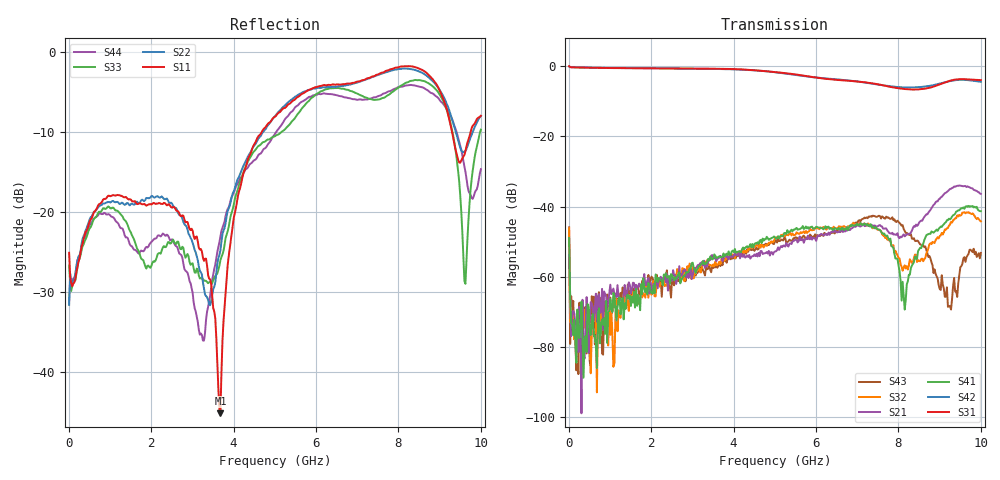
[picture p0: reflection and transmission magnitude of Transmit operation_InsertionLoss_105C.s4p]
! Device:  ADRF5545A
! Description: Dual-Channel, Receiver Front End
! Frequency:  2.4 -  4.2 GHz
! Ports:
!	ANT-CHA	= Port 1
!	ANT-CHB	= Port 2
!  TXOUT-CHA = Port 3
!	TXOUT-CHB = Port 4
! VDD1-CHA, VDD1-CHB, VDD2-CHA, VDD2-CHB, and SWVDD-CHAB = 5 V
! SWCTRL-CHAB = 5 V,  PD-CHAB = 5 V,BP-CHA=BP-CHB=0V
! Temp=105C
! Data:  Data was collected using a calibrated 4 port network analyzer and de-embedded using AtaiTec's In Situ De-Embedding.
! Note:  Analog Devices supplies this data as a sample of measured data
!  for this product.  Your particular data for this product may vary.
!  Data was taken at 105 degrees C.
!  Analog Devices reserves the right to change this data at anytime.
!Correction: S11(Full 4 Port(1,2,3,4))
!S12(Full 4 Port(1,2,3,4))
!S13(Full 4 Port(1,2,3,4))
!S14(Full 4 Port(1,2,3,4))
!S21(Full 4 Port(1,2,3,4))
!S22(Full 4 Port(1,2,3,4))
!S23(Full 4 Port(1,2,3,4))
!S24(Full 4 Port(1,2,3,4))
!S31(Full 4 Port(1,2,3,4))
!S32(Full 4 Port(1,2,3,4))
!S33(Full 4 Port(1,2,3,4))
!S34(Full 4 Port(1,2,3,4))
!S41(Full 4 Port(1,2,3,4))
!S42(Full 4 Port(1,2,3,4))
!S43(Full 4 Port(1,2,3,4))
!S44(Full 4 Port(1,2,3,4))
!S4P File: Measurements: <S11,S12,S13,S14>,
!<S21,S22,S23,S24>,
!<S31,S32,S33,S34>,
!<S41,S42,S43,S44>:
# Hz S  dB  R 50
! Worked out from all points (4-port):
!   401 points, 10 MHz to 10 GHz, reference 50 ohm
!   strongest paths, dB at 10 MHz, 2.507 GHz, 5.005 GHz, 7.503 GHz, 10 GHz:
!     S31: 0.0, -0.7, -1.7, -5.2, -4.0
!     S42: -0.1, -0.7, -1.8, -5.3, -4.5
!     S41: -49.0, -59.5, -48.7, -46.5, -41.3
!     S21: -53.5, -61.1, -52.8, -45.6, -36.4
!     S32: -46.2, -60.0, -49.0, -46.6, -44.2
!     S43: -45.9, -60.5, -49.9, -42.8, -53.2
!   lowest |S11| = -45.2 dB at 3.681 GHz (marker M1), VSWR 1.01, Z = 50.5 - j0.232 ohm
!   |S11| at or under -10 dB: start of sweep to 4.687 GHz; 9.3 GHz to 9.754 GHz (454.1 MHz wide, 4.77 % of centre)
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1e7  -25.12 -82.1  -44.40 131.0  -0.08 -3.4  -48.70 47.9
     -53.54 -105.3  -31.62 -105.9  -57.49 69.1  -0.13 -2.5
     -0.05 -3.7  -46.19 27.7  -26.70 -54.5  -40.96 -49.8
     -48.97 -0.4  -0.15 -2.9  -45.90 73.6  -31.13 -122.3
1.84825e8  -27.53 -62.4  -76.24 152.9  -0.42 -4.6  -77.61 -123.7
           -75.38 144.6  -26.88 -67.8  -74.12 137.6  -0.42 -4.3
           -0.42 -4.6  -75.26 137.8  -27.81 -60.8  -78.47 29.4
           -84.41 53.6  -0.41 -4.3  -86.58 -34.2  -26.93 -64.6
3.681325e9  -45.17 -24.7  -54.51 58.4  -0.81 -86.5  -55.05 -179.5
            -54.01 60.0  -24.79 17.8  -56.14 170.9  -0.87 -82.1
            -0.81 -86.5  -56.43 174.4  -26.03 -118.4  -57.30 -66.9
            -54.36 179.6  -0.85 -82.1  -56.93 -63.8  -23.10 -48.9
5.005e9  -8.12 42.8  -53.31 55.3  -1.74 -124.0  -48.28 129.1
         -52.76 47.6  -8.07 50.4  -48.94 129.5  -1.76 -118.6
         -1.72 -124.0  -49.03 129.3  -10.55 -114.3  -50.19 -173.1
         -48.70 128.3  -1.76 -118.6  -49.94 -175.3  -10.27 -118.1
8.126875e9  -1.82 50.6  -48.40 -38.4  -6.54 169.1  -64.74 -9.3
            -47.91 -37.7  -2.10 55.9  -57.27 -25.4  -6.08 179.5
            -6.53 169.0  -57.30 -19.7  -4.05 89.0  -46.28 -156.4
            -65.28 -9.8  -6.07 179.5  -46.37 -155.0  -4.30 109.3
9.625375e9  -12.43 160.8  -34.02 -148.2  -3.77 122.9  -40.33 -30.2
            -34.16 -148.3  -12.39 146.1  -41.94 -34.0  -3.97 135.1
            -3.77 122.9  -41.91 -34.6  -29.00 -38.7  -55.55 50.7
            -39.99 -30.6  -3.96 135.2  -55.73 57.5  -15.01 32.5
1e10  -8.01 -174.6  -36.39 155.4  -4.02 101.2  -41.54 -82.8
      -36.38 154.5  -8.02 -174.6  -44.03 -85.1  -4.49 113.6
      -4.01 101.2  -44.18 -82.6  -9.72 -96.3  -54.50 -11.4
      -41.31 -83.9  -4.49 113.7  -53.18 -21.8  -14.67 -61.8
